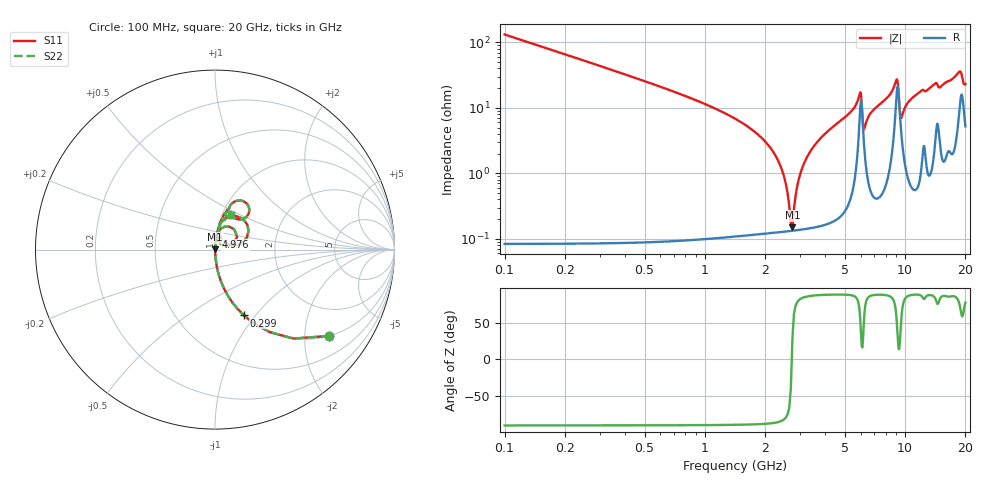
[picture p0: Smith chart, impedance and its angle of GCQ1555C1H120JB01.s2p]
!Murata Part Number: GCQ1555C1H120JB01
!These Parameters are Measured in Series Mode Connection
!Data Generated on Jan 08, 2026
!  o--ll--o
!Port1  Port2
!  o------o
!Operation Temp=25[degC], DC Bias Voltage=0[V]
!Freq. Start=100[MHz] Stop=20[GHz] 401[Steps]
# Hz S RI R 50
!Freq.(Hz) S11(Real) S11(Imag) S21(Real) S21(Imag) S12(Real) S12(Imag) S22(Real) S22(Imag)
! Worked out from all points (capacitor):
!   401 points, 100 MHz to 20 GHz, reference 50 ohm
!   read as one part in series: C = 12 pF near 199.5 MHz
!   lowest |Z| = 150 mohm at 2.737 GHz (marker M1)
!   series resonance near 2.718 GHz, so ESL is about 290 pH
!   S11 on the Smith chart (normalised r, x): 100 MHz: 1.00, -2.65; 299 MHz: 1.00, -0.88; 4.976 GHz: 1.01, +0.14; 20 GHz: 1.10, +0.45
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1e8  0.6368 -0.4806  0.3632 0.4806  0.3632 0.4806  0.6368 -0.4806
2.99e8  0.1616 -0.3671  0.8384 0.3671  0.8384 0.3671  0.1616 -0.3671
8.4625e8  0.0206 -0.1386  0.9794 0.1386  0.9794 0.1386  0.0206 -0.1386
2.1895e9  0.00169 -0.0214  0.9983 0.0214  0.9983 0.0214  0.00169 -0.0214
2.43825e9  0.00139 -0.0107  0.9986 0.0107  0.9986 0.0107  0.00139 -0.0107
2.63725e9  0.00131 -0.00296  0.9987 0.00296  0.9987 0.00296  0.00131 -0.00296
2.73675e9  0.00132 0.000697  0.9987 -0.000697  0.9987 -0.000697  0.00132 0.000697
3.03525e9  0.0015 0.011  0.9985 -0.011  0.9985 -0.011  0.0015 0.011
3.43325e9  0.00202 0.0237  0.998 -0.0237  0.998 -0.0237  0.00202 0.0237
4.9755e9  0.00753 0.0702  0.9925 -0.0702  0.9925 -0.0702  0.00753 0.0702
5.92075e9  0.0773 0.1285  0.9227 -0.1285  0.9227 -0.1285  0.0773 0.1285
6.269e9  0.0231 0.0416  0.9769 -0.0416  0.9769 -0.0416  0.0231 0.0416
6.7665e9  0.012 0.0833  0.988 -0.0833  0.988 -0.0833  0.012 0.0833
8.458e9  0.0392 0.156  0.9608 -0.156  0.9608 -0.156  0.0392 0.156
9.00525e9  0.1399 0.1795  0.8601 -0.1795  0.8601 -0.1795  0.1399 0.1795
9.1545e9  0.1869 0.1043  0.8131 -0.1043  0.8131 -0.1043  0.1869 0.1043
9.50275e9  0.0534 0.0419  0.9466 -0.0419  0.9466 -0.0419  0.0534 0.0419
1.005e10  0.0224 0.1011  0.9776 -0.1011  0.9776 -0.1011  0.0224 0.1011
1.338325e10  0.0489 0.1934  0.9511 -0.1934  0.9511 -0.1934  0.0489 0.1934
1.67165e10  0.0804 0.2341  0.9196 -0.2341  0.9196 -0.2341  0.0804 0.2341
1.87065e10  0.1712 0.2616  0.8288 -0.2616  0.8288 -0.2616  0.1712 0.2616
2e10  0.0915 0.1954  0.9085 -0.1954  0.9085 -0.1954  0.0915 0.1954
